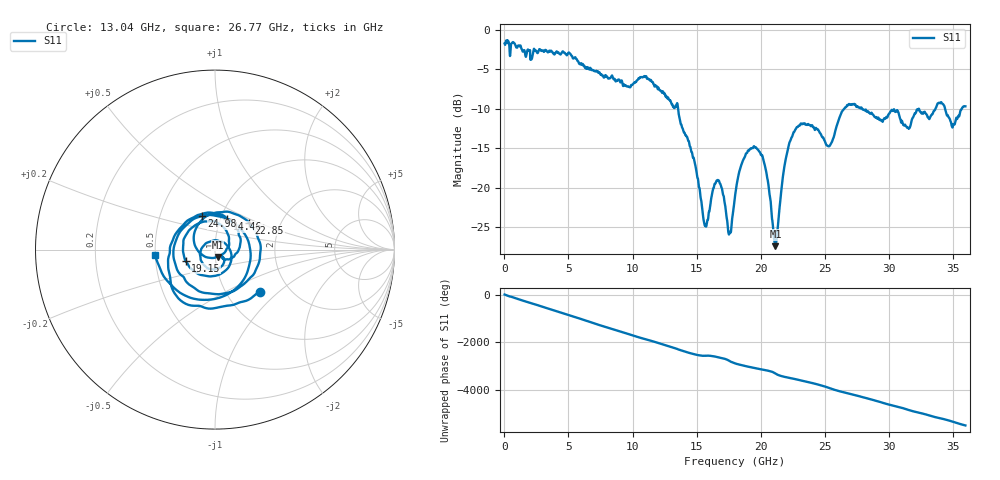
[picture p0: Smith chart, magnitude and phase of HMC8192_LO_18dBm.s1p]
! Analog Devices, Inc.
! 1 Analog Way
! Wilmington, MA 01887
! http://www.analog.com
! Date:  2021-09-17 NN
! Board Name:  EVALHMC8192LG Revision A with HMC8192LG installed
! File Description:  S-Parameters for evaluation board without connectors or board loss de-embedded
! File Generation:  Calibrated Network Analyzer
! Chip Part Number:  HMC8192
! Chip Description:  Wideband IQ Mixer
! Chip Frequency:  20 to 42 GHz
! Chip Package:  LGA_CAV, 4 x 4 x 1.55 mm
! Chip State:
!  Temperature:  25C
!  LO Power:  18dBm
! Note:
!  Analog Devices supplies this data as a sample of measured data at the evaluation board
!  ports for this product.  Your particular data for this product may vary.
!  Analog Devices reserves the right to change this data at anytime.
!  All lines below in this file are as is from the Network Analyzer.
!Keysight Technologies,N5245A,MY49151104,A.10.65.16
!Date: Thursday, September 16, 2021 12:11:29
!Correction: S11(Full 1 Port(1))
!S1P File: Measurement: S11:
# Hz S  dB  R 50
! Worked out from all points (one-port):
!   3600 points, 10 MHz to 36 GHz, reference 50 ohm
!   lowest |S11| = -27.4 dB at 21.16 GHz (marker M1), VSWR 1.09, Z = 51.3 - j4.15 ohm
!   |S11| at or under -10 dB: 13.56 GHz to 26.54 GHz (12.98 GHz wide, 64.7 % of centre); 27.93 GHz to 32.35 GHz (4.418 GHz wide, 14.7 % of centre); 34.41 GHz to 35.71 GHz (1.305 GHz wide, 3.72 % of centre)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
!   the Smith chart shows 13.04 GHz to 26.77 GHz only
!   S11 on the Smith chart (normalised r, x): 13.04 GHz: 1.43, -0.76; 14.46 GHz: 1.08, +0.38; 19.15 GHz: 0.71, -0.09; 22.85 GHz: 1.39, +0.44; 24.98 GHz: 0.81, +0.31; 26.77 GHz: 0.50, -0.04
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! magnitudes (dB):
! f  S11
! 10 MHz  -1.7
! 4.51 GHz  -2.8
! 9.01 GHz  -6.5
! 11.04 GHz  -5.9
! 13.04 GHz  -9.3
! 13.51 GHz  -9.4
! 14.46 GHz  -14.7
! 15.68 GHz  -24.7
! 16.57 GHz  -19.1
! 16.99 GHz  -20.1
! 17.57 GHz  -25.7
! 18.01 GHz  -21.0
! 19.15 GHz  -15.1
! 20.25 GHz  -16.7
! 21.16 GHz  -27.4
! 21.89 GHz  -17.0
! 22.51 GHz  -13.3
! 22.85 GHz  -12.3
! 24.98 GHz  -14.0
! 25.47 GHz  -14.5
! 26.77 GHz  -9.5
! 27.01 GHz  -9.5
! 29.42 GHz  -11.4
! 30.57 GHz  -10.4
! 31.51 GHz  -12.4
! 34 GHz  -9.3
! 35.05 GHz  -12.0
! 36 GHz  -9.7
